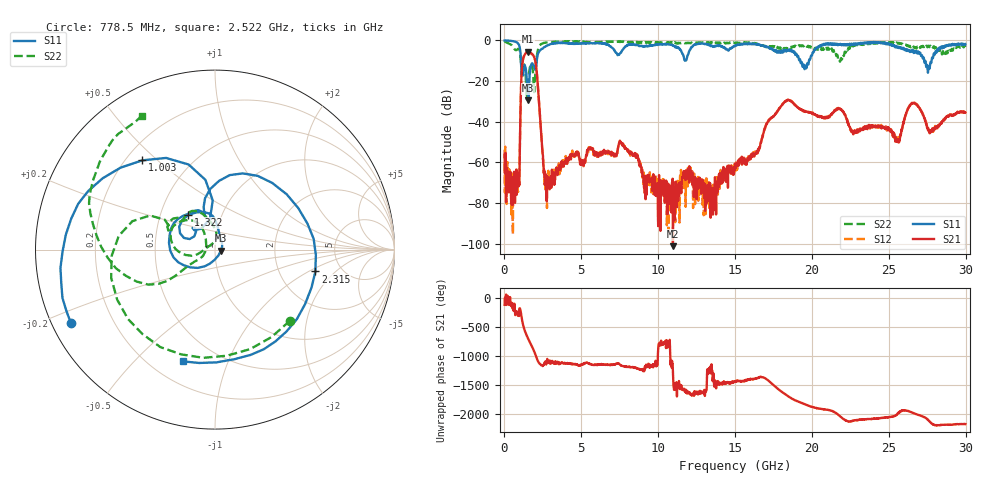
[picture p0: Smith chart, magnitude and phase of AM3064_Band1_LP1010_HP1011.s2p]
# Hz S DB R 50.0
!freq dBS11 angS11 dBS21 angS21 dBS12 angS12 dBS22 angS22
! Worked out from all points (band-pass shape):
!   1600 points, 10 MHz to 29.98 GHz, reference 50 ohm
!   highest |S21| = -5.54 dB at 1.528 GHz (marker M1); lowest = -101.3 dB at 10.96 GHz (marker M2)
!   |S21| within 3 dB of the highest: 1.234 GHz to 1.947 GHz (713.3 MHz wide, 44.9 % of centre)
!   lowest |S11| = -29.5 dB at 1.547 GHz (marker M3), VSWR 1.07, Z = 53.4 - j0.649 ohm
!   |S11| at or under -10 dB: 1.071 GHz to 2.101 GHz (1.03 GHz wide, 64.9 % of centre); 19.25 GHz to 19.81 GHz (561.6 MHz wide, 2.88 % of centre); 27.3 GHz to 27.78 GHz (479.2 MHz wide, 1.74 % of centre)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
!   |S22| runs from -29.0 to -0.4 dB; largest |S21 - S12| = 0.0076
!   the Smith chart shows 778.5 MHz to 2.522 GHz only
!   S11 on the Smith chart (normalised r, x): 778.5 MHz: 0.06, -0.24; 1.003 GHz: 0.26, +0.45; 1.322 GHz: 0.69, +0.29; 2.315 GHz: 3.22, -1.16; 2.522 GHz: 0.33, -0.70
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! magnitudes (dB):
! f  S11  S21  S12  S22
! 10 MHz  0.0  -56.2  -53.8  -0.4
! 778.5 MHz  -0.9  -63.5  -67.6  -4.8
! 1.003 GHz  -3.9  -51.4  -51.2  -5.3
! 1.172 GHz  -15.5  -11.0  -10.9  -11.2
! 1.322 GHz  -12.3  -7.0  -6.9  -12.6
! 1.528 GHz  -27.2  -5.5  -5.5  -20.0
! 1.547 GHz  -29.5  -5.6  -5.5  -18.6
! 1.997 GHz  -14.4  -9.8  -9.7  -17.5
! 2.315 GHz  -4.8  -37.8  -37.6  -2.3
! 2.522 GHz  -3.8  -60.9  -58.7  -1.4
! 2.859 GHz  -2.3  -67.3  -64.1  -0.9
! 5.015 GHz  -1.4  -61.1  -59.3  -0.6
! 7.582 GHz  -6.0  -50.3  -50.0  -0.5
! 10 GHz  -2.0  -91.4  -73.3  -1.0
! 10.96 GHz  -2.3  -101.3  -74.3  -1.1
! 15 GHz  -2.7  -60.7  -61.4  -1.3
! 18.29 GHz  -4.6  -30.1  -29.9  -3.9
! 19.99 GHz  -7.5  -35.9  -35.7  -3.2
! 25 GHz  -1.5  -42.9  -43.1  -1.1
! 26.61 GHz  -6.1  -30.8  -30.8  -3.0
! 27.56 GHz  -15.0  -43.5  -43.5  -2.7
! 29.98 GHz  -1.8  -35.5  -35.3  -3.2
